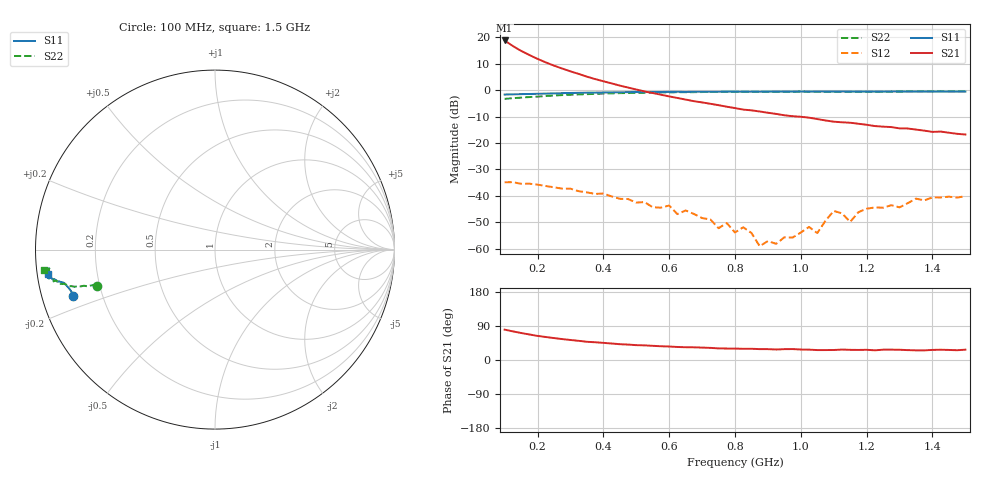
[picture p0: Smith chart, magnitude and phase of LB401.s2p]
!  POLYFET RF DEVICES
!  LB401 (Each Side)
!  S PARAMETERS
!  VDS=28V, IDQ=600mA
! Date: Wed Apr 07 15:05:08 1999
! SCATTERING PARAMETERS :
# MHZ S MA R 50
! Freq=Mhz Mag[s11] Ang[s11] Mag[s21] Ang[s21] Mag[s12] Ang[s12] Mag[s22] Ang[s22]
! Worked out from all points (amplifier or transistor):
!   57 points, 100 MHz to 1.5 GHz, reference 50 ohm
!   highest |S21| = 18.8 dB at 100 MHz (marker M1)
!   |S21| within 3 dB of that: start of sweep to 137.2 MHz
!   unconditionally stable (mu >= 1): 483.2 MHz to end of sweep
!   at 325 MHz: K = 0.52, MSG = 22.2 dB, |S12| = -38.2 dB
!   at 800 MHz: K = 7.86, MAG = 11.6 dB, |S12| = -53.9 dB
!   at 1.5 GHz: K = 3.81, MAG = 2.9 dB, |S12| = -40.1 dB
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100  0.829 -162.0  8.744 80.2  0.01813 -7.5  0.6874 -163.0
125  0.8351 -164.0  6.865 75.6  0.0182 -10.3  0.7067 -163.7
150  0.8432 -165.4  5.554 71.3  0.01698 -14.0  0.7245 -163.9
175  0.8492 -166.1  4.641 67.4  0.01705 -16.7  0.7423 -164.0
200  0.8562 -167.2  3.919 63.6  0.01636 -23.1  0.7567 -164.6
250  0.8706 -168.0  2.919 57.9  0.01456 -24.4  0.7939 -165.1
350  0.8993 -168.9  1.806 48.1  0.01167 -32.9  0.8424 -166.1
450  0.9146 -169.7  1.224 41.7  0.00882 -38.2  0.8816 -167.5
575  0.9263 -170.6  0.822 36.3  0.006 -35.8  0.9066 -168.9
650  0.929 -170.4  0.6656 33.7  0.00531 -22.3  0.9155 -169.6
750  0.9366 -171.0  0.5215 30.6  0.00245 -15.2  0.9287 -170.6
775  0.9398 -170.8  0.4876 30.3  0.00307 -16.5  0.9274 -170.8
800  0.9384 -170.6  0.4595 30.1  0.00203 -31.8  0.9298 -171.1
825  0.9373 -170.1  0.43 29.6  0.00255 -20.3  0.9305 -171.5
875  0.9381 -171.0  0.3959 28.7  0.00112 -79.4  0.9343 -171.8
1025  0.9405 -170.8  0.3025 27.4  0.00259 122.1  0.9353 -173.0
1050  0.9463 -171.2  0.2847 26.2  0.00198 122.3  0.9341 -173.0
1100  0.9449 -171.8  0.2541 26.4  0.0052 109.8  0.9304 -173.5
1150  0.9442 -171.1  0.2425 26.8  0.00323 111.4  0.9324 -173.5
1200  0.9435 -171.9  0.2218 27.0  0.00572 119.8  0.9315 -173.4
1275  0.9459 -172.4  0.2009 27.3  0.00668 116.9  0.9394 -173.1
1500  0.9411 -171.5  0.1452 27.3  0.00989 119.7  0.9589 -173.3
